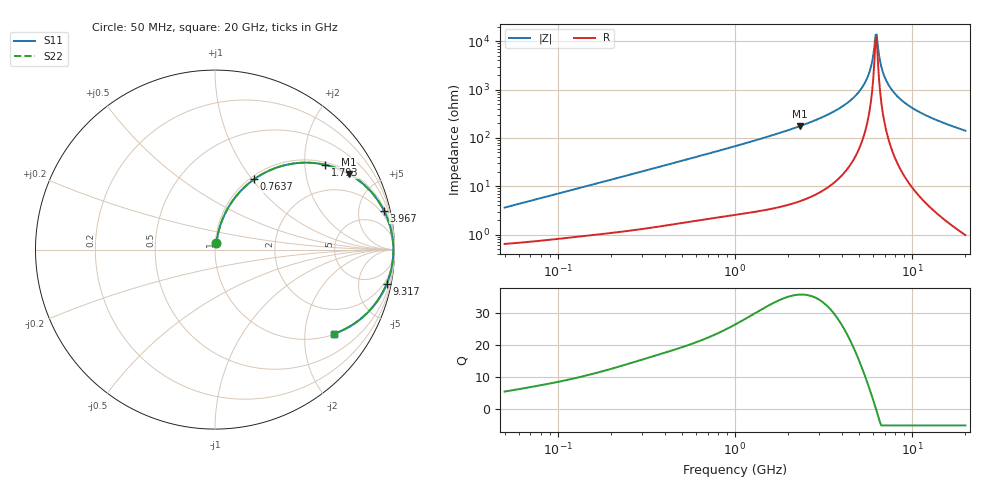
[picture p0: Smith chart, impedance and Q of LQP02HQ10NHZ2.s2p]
!Murata Part Number: LQP02HQ10NHZ2
!These Parameters are Measured in Series Mode Connection
!  o--[Z]--o
!Port1  Port2
!  o-------o
!Freq. Start=50[MHz] Stop=20[GHz], 401[Steps]
# Hz S RI R 50
!Freq.(Hz) S11(Real) S11(Imag) S21(Real) S21(Imag) S12(Real) S12(Imag) S22(Real) S22(Imag)
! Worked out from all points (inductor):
!   401 points, 50 MHz to 20 GHz, reference 50 ohm
!   read as one part in series: L = 11.3 nH near 51.52 MHz
!   highest Q = 35.8 at 2.314 GHz (marker M1), where L = 12 nH
!   self-resonance near 6.218 GHz
!   S11 on the Smith chart (normalised r, x): 50 MHz: 1.01, +0.07; 763.7 MHz: 1.04, +1.02; 1.793 GHz: 1.07, +2.54; 3.967 GHz: 1.32, +8.58; 9.317 GHz: 1, -10; 20 GHz: 1.02, -2.82
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5e7  0.00761 0.0351  0.9924 -0.0351  0.9924 -0.0351  0.00761 0.0351
1.364002e8  0.0177 0.0917  0.9823 -0.0917  0.9823 -0.0917  0.0177 0.0917
3.721004e8  0.0711 0.2295  0.9289 -0.2295  0.9289 -0.2295  0.0711 0.2295
7.636728e8  0.2174 0.3915  0.7826 -0.3915  0.7826 -0.3915  0.2174 0.3915
1e9  0.3185 0.4474  0.6815 -0.4474  0.6815 -0.4474  0.3185 0.4474
1.793498e9  0.615 0.4722  0.385 -0.4722  0.385 -0.4722  0.615 0.4722
2.313601e9  0.7462 0.4215  0.2538 -0.4215  0.2538 -0.4215  0.7462 0.4215
2.728004e9  0.8202 0.3701  0.1798 -0.3701  0.1798 -0.3701  0.8202 0.3701
3.967106e9  0.9413 0.2171  0.0587 -0.2171  0.0587 -0.2171  0.9413 0.2171
4.748272e9  0.9742 0.1336  0.0258 -0.1336  0.0258 -0.1336  0.9742 0.1336
5.352748e9  0.9872 0.0763  0.0128 -0.0763  0.0128 -0.0763  0.9872 0.0763
5.769027e9  0.9918 0.0401  0.00821 -0.0401  0.00821 -0.0401  0.9918 0.0401
5.944466e9  0.9929 0.0256  0.00714 -0.0256  0.00714 -0.0256  0.9929 0.0256
6.125241e9  0.9935 0.0111  0.0065 -0.0111  0.0065 -0.0111  0.9935 0.0111
6.217679e9  0.9937 0.00379  0.00634 -0.00379  0.00634 -0.00379  0.9937 0.00379
6.406762e9  0.9936 -0.0108  0.00635 0.0108  0.00635 0.0108  0.9936 -0.0108
6.701223e9  0.9928 -0.0326  0.00718 0.0326  0.00718 0.0326  0.9928 -0.0326
6.905011e9  0.9917 -0.0471  0.00827 0.0471  0.00827 0.0471  0.9917 -0.0471
7.442007e9  0.9871 -0.0834  0.0129 0.0834  0.0129 0.0834  0.9871 -0.0834
9.316812e9  0.9566 -0.1906  0.0434 0.1906  0.0434 0.1906  0.9566 -0.1906
1.295331e10  0.865 -0.3353  0.135 0.3353  0.135 0.3353  0.865 -0.3353
2e10  0.6649 -0.4686  0.3351 0.4686  0.3351 0.4686  0.6649 -0.4686
